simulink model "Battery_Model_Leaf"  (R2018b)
settings: Solver=VariableStepAuto  StartTime=0.0  StopTime=1369  FixedStep=1e-3  RelTol=1e-5
libraries: fl_lib x10, nesl_utility x10, elec_lib x3

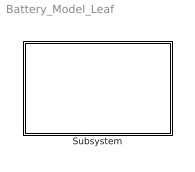
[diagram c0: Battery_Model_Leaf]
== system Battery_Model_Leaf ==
  Subsystem : Subsystem

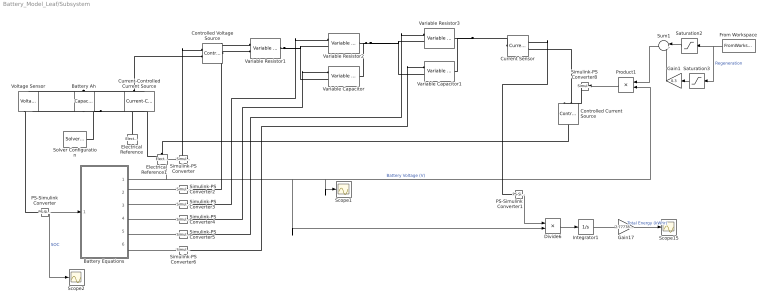
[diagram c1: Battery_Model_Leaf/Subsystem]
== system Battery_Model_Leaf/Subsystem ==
  Battery Ah : elec_lib/Passive Devices/Capacitor  enable_table=0  c=400000 F  Cvec=[1e-05, 1e-06] F  Vvec=[0, 10] V  CV_table_symmetry=1  C_tol=0  enable_C_tol=0  tol_distribution=1  nSigma=4  r=1e-6 Ohm  g=0 1/Ohm  enable_operating_limits=0  operating_limit_action=2  max_working_voltage_range=[-25, 25] V  power_rating=1 W  enable_faults=0  fault_action=1  Cscale_faulted=100  R_faulted=1e-3 Ohm  G_faulted=0 1/Ohm  tau_fault=1e-3 s  enable_temporal_fault=0  t_fault=1 s  enable_behavioral_fault=0  max_permissible_voltage_range=[-100, 100] V  t_fail_on_voltage=1 s  i_specify=off  i_priority=None  i=0 A  i_nominal_specify=off  i_nominal_unit=A  i_nominal_value=1  v_specify=off  v_priority=None  v=1 V  v_nominal_specify=off  v_nominal_unit=V  v_nominal_value=1  vc_specify=on  vc_priority=High  vc=1 V  vc_nominal_specify=off  vc_nominal_unit=V  vc_nominal_value=1
  Battery Equations : MATLAB Function  TreatAsAtomicUnit=on
  Controlled Current Source : fl_lib/Electrical/Electrical Sources/Controlled Current Source
  Controlled Voltage Source : fl_lib/Electrical/Electrical Sources/Controlled Voltage Source
  Current Sensor : fl_lib/Electrical/Electrical Sensors/Current Sensor
  Current-Controlled Current Source : fl_lib/Electrical/Electrical Sources/Current-Controlled Current Source  K=1  i1_specify=off  i1_priority=None  i1=0 A  i1_nominal_specify=off  i1_nominal_unit=A  i1_nominal_value=1  i2_specify=off  i2_priority=None  i2=0 A  i2_nominal_specify=off  i2_nominal_unit=A  i2_nominal_value=1
  Divide6 : Product  Inputs=**
  Electrical Reference : fl_lib/Electrical/Electrical Elements/Electrical Reference
  Electrical Reference1 : fl_lib/Electrical/Electrical Elements/Electrical Reference
  From Workspace : FromWorkspace  VariableName=Battery_Power_Leaf  SampleTime=0
  Gain1 : Gain  Gain=0.3
  Gain17 : Gain  Gain=2.77778e-7
  Integrator1 : Integrator
  PS-Simulink Converter : nesl_utility/PS-Simulink Converter  PhysicalDomain=network_engine_domain  SubClassName=ps_output  LeftPortType=input  RightPortType=output  PseudoPeriodic=off  Frequencies=[]  Unit=1  AffineConversion=off
  PS-Simulink Converter1 : nesl_utility/PS-Simulink Converter  PhysicalDomain=network_engine_domain  SubClassName=ps_output  LeftPortType=input  RightPortType=output  PseudoPeriodic=off  Frequencies=[]  Unit=1  AffineConversion=off
  Product1 : Product  Inputs=*/
  Saturation2 : Saturate  UpperLimit=inf  LowerLimit=0
  Saturation3 : Saturate  UpperLimit=0  LowerLimit=-inf
  Scope1 : Scope
  Scope15 : Scope
  Scope2 : Scope
  Simulink-PS Converter{,2..6,8} (7 alike) : nesl_utility/Simulink-PS Converter  PhysicalDomain=network_engine_domain  SubClassName=ps_input  LeftPortType=input  RightPortType=output  PseudoPeriodic=off  Frequencies=[]  NoiseDistribution=none  NoiseParameters=[]  Unit=1  AffineConversion=off  FilteringAndDerivatives=provide  SimscapeFilterOrder=1  InputFilterTimeConstant=0.001  UdotUserProvided=0
  Solver Configuration : nesl_utility/Solver Configuration  PhysicalDomain=network_engine_domain  SubClassName=solver  LeftPortType=input  RightPortType=generic  Tones=[]  Harmonics=[]  SimulateNoise=off  Profile=off  UseLocalSampling=off  EnableSwitchedLinearOptims=on  FrequencyDomain=off  UseCCode=off  RelTol=0.001  AbsTol=1e-06  MinStep=1e-09  ToWorkspace=off  RevertToSquareIcSolve=off  NumHomotopyIterations=100  PhasorMode=off  PhasorModeNumHarmonics=1  DoDC=off  ResidualTolerance=1e-09  UseLocalSolver=off  LocalSolverChoice=NE_BACKWARD_EULER_ADVANCER  LocalSolverSampleTime=0.001  DoFixedCost=off  MaxNonlinIter=3  MaxModeIter=2  LinearAlgebra=auto  EquationFormulation=NE_TIME_EF  DelaysMemoryBudget=1024  AutomaticFiltering=on  FilteringTimeConstant=0.001  PartitionStorageMethod=AS_NEEDED  PartitionMemoryBudget=1024
  Sum1 : Sum  Inputs=|++
  Variable Capacitor : elec_lib/Passive Devices/Variable Capacitor  prm=2  Cmin=1e-9 F  r=1e-6 Ohm  v0=0 V  q0=0 C
  Variable Capacitor1 : elec_lib/Passive Devices/Variable Capacitor  prm=2  Cmin=1e-9 F  r=1e-6 Ohm  v0=0 V  q0=0 C
  Variable Resistor1 : fl_lib/Electrical/Electrical Elements/Variable Resistor  Rmin=0 Ohm  i_specify=off  i_priority=None  i=0 A  i_nominal_specify=off  i_nominal_unit=A  i_nominal_value=1  v_specify=off  v_priority=None  v=0 V  v_nominal_specify=off  v_nominal_unit=V  v_nominal_value=1
  Variable Resistor2 : fl_lib/Electrical/Electrical Elements/Variable Resistor  Rmin=0 Ohm  i_specify=off  i_priority=None  i=0 A  i_nominal_specify=off  i_nominal_unit=A  i_nominal_value=1  v_specify=off  v_priority=None  v=0 V  v_nominal_specify=off  v_nominal_unit=V  v_nominal_value=1
  Variable Resistor3 : fl_lib/Electrical/Electrical Elements/Variable Resistor  Rmin=0 Ohm  i_specify=off  i_priority=None  i=0 A  i_nominal_specify=off  i_nominal_unit=A  i_nominal_value=1  v_specify=off  v_priority=None  v=0 V  v_nominal_specify=off  v_nominal_unit=V  v_nominal_value=1
  Voltage Sensor : fl_lib/Electrical/Electrical Sensors/Voltage Sensor
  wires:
  PS-Simulink Converter/1 -> Battery Equations/1(Soc), Scope2/1  "SOC"
  Battery Equations/1(Voc) -> Divide6/2, Scope1/1, Product1/2, Simulink-PS Converter/1  "Battery Voltage (V)"
  Battery Equations/2(Rs) -> Simulink-PS Converter2/1
  Battery Equations/3(Rts) -> Simulink-PS Converter3/1
  Battery Equations/4(Cts) -> Simulink-PS Converter4/1
  Battery Equations/5(Rtl) -> Simulink-PS Converter5/1
  Battery Equations/6(Ctl) -> Simulink-PS Converter6/1
  PS-Simulink Converter1/1 -> Divide6/1
  Divide6/1 -> Integrator1/1
  Integrator1/1 -> Gain17/1
  From Workspace/1 -> Saturation3/1, Saturation2/1  "Regeneration"
  Product1/1 -> Simulink-PS Converter8/1
  Saturation2/1 -> Sum1/1
  Saturation3/1 -> Gain1/1
  Gain1/1 -> Sum1/2
  Sum1/1 -> Product1/1
  Gain17/1 -> Scope15/1  "Total Energy (kWhr)"
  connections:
  Controlled Voltage Source/LConn1 -- Variable Resistor1/LConn2
  Variable Resistor2/RConn1 -- Variable Resistor3/LConn2 -- Variable Capacitor1/LConn2 -- Variable Capacitor/RConn1
  Battery Ah/LConn1 -- Current-Controlled Current Source/RConn2 -- Voltage Sensor/LConn1
  Battery Ah/RConn1 -- Solver Configuration/RConn1 -- Electrical Reference/LConn1 -- Current-Controlled Current Source/LConn2 -- Voltage Sensor/RConn2
  Variable Resistor1/RConn1 -- Variable Capacitor/LConn2 -- Variable Resistor2/LConn2
  Current Sensor/LConn1 -- Variable Capacitor1/RConn1 -- Variable Resistor3/RConn1
  Electrical Reference1/LConn1 -- Controlled Current Source/LConn1 -- Current-Controlled Current Source/LConn1
  Current-Controlled Current Source/RConn1 -- Controlled Voltage Source/RConn2
  Voltage Sensor/RConn1 -- PS-Simulink Converter/LConn1
  Simulink-PS Converter/RConn1 -- Controlled Voltage Source/RConn1
  Simulink-PS Converter2/RConn1 -- Variable Resistor1/LConn1
  Simulink-PS Converter3/RConn1 -- Variable Resistor2/LConn1
  Simulink-PS Converter4/RConn1 -- Variable Capacitor/LConn1
  Simulink-PS Converter5/RConn1 -- Variable Resistor3/LConn1
  Simulink-PS Converter6/RConn1 -- Variable Capacitor1/LConn1
  Controlled Current Source/RConn2 -- Current Sensor/RConn2
  PS-Simulink Converter1/LConn1 -- Current Sensor/RConn1
  Simulink-PS Converter8/RConn1 -- Controlled Current Source/RConn1

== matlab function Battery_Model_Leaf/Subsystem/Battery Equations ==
function [Voc,Rs,Rts,Cts,Rtl,Ctl] = fcn(Soc)
Voc=360/375*91.4*(-1.031*exp(-35*Soc)+3.685+0.2156*Soc-0.1178*Soc^2+0.3201*Soc^3);
Rs=360/375*91.4*(0.1562*exp(-24.37*Soc)+0.07446);
Rts=0.3208*exp(-29.14*Soc)+0.04669;
Cts=-752.9*exp(-13.51*Soc)+703.6;
Rtl=6.603*exp(-155.2*Soc)+0.04984;
Ctl=-6056*exp(-27.12*Soc)+4475;
end
